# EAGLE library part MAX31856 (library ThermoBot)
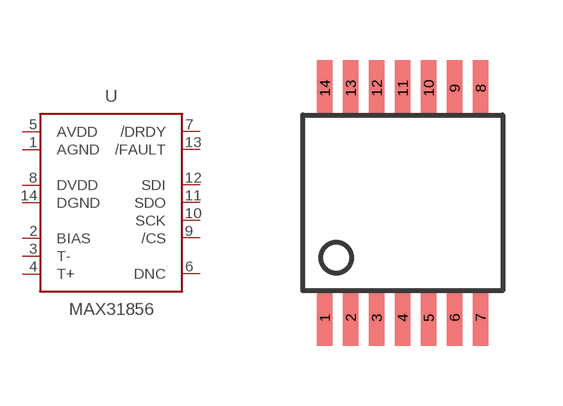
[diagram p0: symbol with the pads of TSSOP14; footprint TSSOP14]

Designator prefix -

## MAX31856 (MPN: MAX31856MUD+; PN-DK: MAX31856MUD+-ND)  [TSSOP14]
1  AGND  pwr
2  BIAS
3  T-
4  T+
5  AVDD  pwr
6  DNC  nc
7  /DRDY
8  DVDD  pwr
9  /CS
10  SCK
11  SDO
12  SDI
13  /FAULT
14  DGND  pwr

## Footprint TSSOP14 (pad centres in mm)
smd 0.38 x 1.4: 1 -1.95,-2.875; 2 -1.3,-2.875; 3 -0.65,-2.875; 4 0,-2.875; 5 0.65,-2.875; 6 1.3,-2.875; 7 1.95,-2.875; 8 1.95,2.875; 9 1.3,2.875; 10 0.65,2.875; 11 0,2.875; 12 -0.65,2.875; 13 -1.3,2.875; 14 -1.95,2.875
